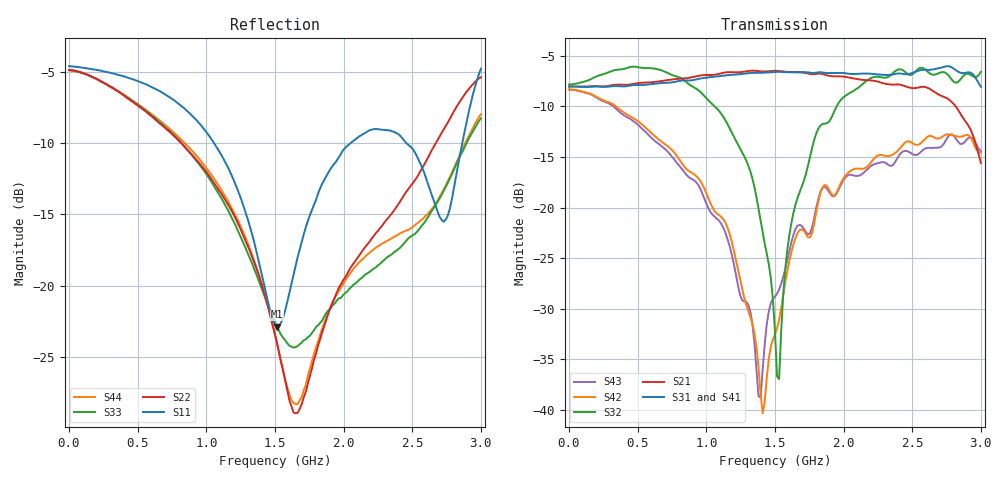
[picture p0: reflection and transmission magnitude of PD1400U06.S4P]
!Agilent Technologies,E5071C,MY46103565,A.11.31
!Date: Fri Mar 24 03:21:09 2017
!Data & Calibration Information:
!Freq	S11:SOLT4(ON)	S12:SOLT4(ON)	S13:SOLT4(ON)	S14:SOLT4(ON)
!	S21:SOLT4(ON)	S22:SOLT4(ON)	S23:SOLT4(ON)	S24:SOLT4(ON)
!	S31:SOLT4(ON)	S32:SOLT4(ON)	S33:SOLT4(ON)	S34:SOLT4(ON)
!	S41:SOLT4(ON)	S42:SOLT4(ON)	S43:SOLT4(ON)	S44:SOLT4(ON)
!PortZ  Port1:50+j0  Port2:50+j0  Port3:50+j0  Port4:50+j0
!Above PortZ is port z conversion or system Z0 setting when saving the data.
!When reading, reference impedance value at option line is always used.
# Hz S dB R 50
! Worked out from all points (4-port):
!   201 points, 1 MHz to 3 GHz, reference 50 ohm
!   strongest paths, dB at 1 MHz, 750.8 MHz, 1.5 GHz, 2.25 GHz, 3 GHz:
!     S31: -8.0, -7.6, -6.6, -6.8, -8.1
!     S41: -8.0, -7.5, -6.6, -7.0, -8.8
!     S21: -8.0, -7.3, -6.5, -7.5, -15.6
!     S32: -7.8, -6.9, -32.3, -7.1, -6.6
!     S42: -8.3, -14.3, -32.6, -14.8, -14.6
!     S43: -8.3, -15.0, -28.8, -15.6, -14.4
!   lowest |S11| = -22.9 dB at 1.515 GHz (marker M1), VSWR 1.16, Z = 44.9 - j4.5 ohm
!   |S11| at or under -10 dB: 1.056 GHz to 2.052 GHz (995.3 MHz wide, 64.1 % of centre); 2.456 GHz to 2.865 GHz (408.2 MHz wide, 15.3 % of centre)
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1000000  -4.62 179.9  -8.01 -0.1  -8.02 -0.2  -8.02 -0.2
         -8.03 -0.1  -4.88 179.7  -7.82 -0.1  -8.30 -0.3
         -8.03 -0.2  -7.83 -0.1  -4.90 179.7  -8.32 -0.2
         -8.03 -0.1  -8.32 -0.2  -8.33 -0.3  -4.90 179.7
1.11063e9  -10.85 7.6  -6.88 -155.0  -7.02 -157.1  -7.13 -155.3
           -6.71 -154.1  -13.57 -92.1  -10.71 -145.5  -21.00 140.5
           -6.97 -156.5  -10.76 -146.3  -13.88 -93.6  -21.72 164.4
           -6.95 -154.6  -20.96 140.8  -21.64 164.8  -13.31 -89.8
1.41053e9  -19.45 -71.8  -6.50 157.3  -6.68 155.8  -6.63 157.7
           -6.54 157.1  -20.13 -177.0  -22.43 177.2  -41.90 -13.1
           -6.67 155.6  -22.51 177.0  -20.39 169.8  -35.94 -134.0
           -6.66 157.5  -40.36 -8.1  -36.07 -133.2  -20.06 -175.7
1.515495e9  -22.86 -136.0  -6.49 140.1  -6.56 138.7  -6.58 140.8
            -6.48 139.8  -24.02 143.5  -36.41 -142.8  -31.70 -120.6
            -6.58 138.5  -36.72 -146.1  -22.86 123.7  -28.49 -135.3
            -6.58 140.4  -31.94 -120.9  -28.52 -134.8  -24.02 144.3
1.83039e9  -13.13 95.8  -7.15 85.8  -6.99 84.5  -7.16 88.1
           -6.75 87.3  -23.71 -41.8  -11.89 -88.7  -18.69 -169.6
           -6.61 86.4  -11.91 -88.5  -22.58 -21.6  -18.59 -164.2
           -6.67 88.9  -18.60 -169.0  -18.48 -164.3  -23.38 -36.6
2.475175e9  -10.16 -22.5  -7.71 -20.3  -6.57 -18.3  -6.28 -16.3
            -8.12 -27.7  -13.17 -162.3  -6.92 174.9  -13.65 60.7
            -6.79 -23.4  -6.86 175.8  -16.64 -162.3  -14.53 76.4
            -6.75 -19.3  -13.45 60.6  -14.49 75.0  -16.06 -161.4
3e9  -4.80 -25.3  -15.11 -161.7  -7.25 -135.1  -8.07 -134.7
     -15.58 -172.3  -5.39 103.2  -6.49 131.4  -14.57 -53.7
     -8.06 -140.4  -6.57 131.3  -8.27 126.8  -14.36 -32.4
     -8.76 -139.0  -14.58 -53.8  -14.42 -31.8  -7.98 138.9
